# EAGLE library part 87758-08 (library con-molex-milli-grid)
HEADER
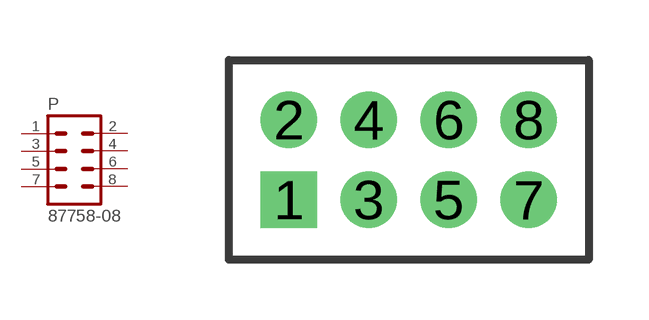
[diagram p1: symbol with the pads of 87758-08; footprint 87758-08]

Designator prefix P

## 87758-08  [87758-08]
1  1  pas
2  2  pas
3  3  pas
4  4  pas
5  5  pas
6  6  pas
7  7  pas
8  8  pas

## Footprint 87758-08 (pad centres in mm)
HEADER Dual Row, Vertical
drill 0.914 square: 1 -3,-1
drill 0.914: 2 -3,1; 3 -1,-1; 4 -1,1; 5 1,-1; 6 1,1; 7 3,-1; 8 3,1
